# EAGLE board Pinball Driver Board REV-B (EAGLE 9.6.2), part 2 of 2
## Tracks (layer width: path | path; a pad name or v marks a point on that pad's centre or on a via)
+3.3VDC
  Top 1.016: R87.2 52.07,109.86
  Top 2.032: U$1.OUT C46.+ 49.53,109.86 52.07,109.86 179.07,109.86 209.66,140.44 209.66,153.03 | X12.1 209.66,153.03 | X6.1 247.12,153.78 246.38,153.03 | 209.66,153.03 246.38,153.03 | X11.3 296.32,155.99 293.37,153.03 246.38,153.03
+12VDC
  Top 0.406: 45.01,165.33 44.86,165.33 45.01,167.81
  Top 1.016: R73.2 45.01,156.84 | ARDUINO_DUE_MASTER.VIN 299.8,100.97 311.15,112.31 311.15,130.18 324.22,143.25 X26.1
  Top 2.032: X26.1 334.24,148.56 334.24,148.59 | 45.01,167.88 45.01,167.81 45.01,165.33 X25.1 45.01,156.84 42.47,154.31 42.47,121.24 39.34,118.11 C45.+ 38.73,117.48 U$1.IN | X11.5 304.24,167.25 304.8,167.81
  Top 2.54: X8.5 22.22,155.58 X8.6
  Top 5.08: 22.22,155.58 22.22,158.36 31.75,167.88 45.01,167.88 | 45.01,167.81 304.8,167.81 320.11,167.81 334.24,153.67 334.24,148.59
/LATCHSEL0  (via drill 0.35)
  Top 0.406: v224.08,111.68 207.82,111.68 IC8.14
  Bottom 0.406: v224.08,111.68 224.49,111.28 224.49,75.51 226.92,73.08 226.92,53.98 226.11,53.16 221.23,53.16 221.23,60.88 217.17,64.95 IC9.4
/LATCHSEL1
  Top 0.406: IC10.14 207.82,84.45 210.26,82.02 218.8,82.02 220.01,80.8 220.01,62.51 217.17,62.51 IC9.5
/LATCHSEL2
  Top 0.406: IC11.14 207.82,57.23 210.26,59.67 217.17,59.67 IC9.6
/LATCHSEL3  (via drill 0.35)
  Top 0.406: v218.8,34.06 211.89,34.06 207.82,30 IC12.14
  Bottom 0.406: v218.8,34.06 218.8,53.57 219.2,53.98 219.2,55.19 217.17,57.23 IC9.7
/WRITETOCOIL  (via drill 0.35)
  Top 0.406: v218.8,80.39 218.8,74.3 217.17,72.67 IC9.1 | v218.8,104.78 250.09,104.78 ARDUINO_DUE_MASTER.8
  Bottom 0.406: v218.8,104.78 v218.8,80.39
A0  (via drill 0.35)
  Top 0.406: v293.17,106.4 296.01,106.4 296.01,101.52 295.2,100.71 284.63,100.71 284.63,96.65 285.44,95.83 298.45,95.83 ARDUINO_DUE_MASTER.A0 | v293.17,141.35 285.44,149.07 272.03,149.07 v270.81,150.29
  Bottom 0.406: v293.17,141.35 v293.17,106.4 | v270.81,150.29 270.81,159.64 X6.7
A1  (via drill 0.35)
  Top 0.406: v286.26,127.53 v300.48,127.53 | v286.26,141.35 279.35,148.26 268.38,148.26 v267.16,149.48
  Bottom 0.406: v300.48,127.53 300.89,127.13 300.89,95.83 298.45,93.4 ARDUINO_DUE_MASTER.A1 | v286.26,141.35 v286.26,127.53 | v267.16,149.48 267.16,159.64 X6.6
A2  (via drill 0.35)
  Top 0.406: v301.3,141.35 292.35,150.29 v272.44,150.29
  Bottom 0.406: v301.3,141.35 301.3,131.19 299.26,129.16 299.26,127.13 300.08,126.31 300.08,100.31 296.82,97.05 296.82,92.58 298.45,90.96 ARDUINO_DUE_MASTER.A2 | v272.44,150.29 270.41,148.26 263.09,148.26 263.09,159.64 X6.5
A3  (via drill 0.35)
  Top 0.406: v294.79,103.15 290.32,107.62 286.66,107.62 v286.26,107.21 | v283.41,141.35 283.41,141.76 278.54,146.63 260.65,146.63 v259.03,148.26
  Bottom 0.406: v294.79,103.15 295.2,103.15 296.01,102.34 296.01,90.96 298.45,88.52 ARDUINO_DUE_MASTER.A3 | v286.26,107.21 284.23,109.25 284.23,137.69 283.41,138.51 v283.41,141.35 | v259.03,148.26 259.03,159.64 X6.4
A4  (via drill 0.35)
  Top 0.406: v302.92,86.08 298.45,86.08 ARDUINO_DUE_MASTER.A4 | v303.73,129.97 299.26,129.97 298.86,129.56 276.1,129.56 v275.69,129.97 | v275.69,141.35 272.03,145.01 258.22,145.01 v254.96,148.26
  Bottom 0.406: v302.92,86.08 303.33,86.49 303.33,129.56 v303.73,129.97 | v275.69,141.35 v275.69,129.97 | v254.96,148.26 254.96,159.64 X6.3
A5  (via drill 0.35)
  Top 0.406: v294.79,101.93 289.51,101.93 v285.04,106.4 | v282.19,141.35 277.72,145.82 259.03,145.82 255.37,149.48 v251.31,149.48
  Bottom 0.406: v294.79,101.93 294.79,86.89 298.45,83.24 ARDUINO_DUE_MASTER.A5 | v285.04,106.4 283.41,108.03 283.41,137.29 282.19,138.51 v282.19,141.35 | v251.31,149.48 251.31,159.64 X6.2
A6  (via drill 0.35)
  Top 0.406: v284.63,138.91 v302.51,138.91 | v284.63,141.35 284.63,141.76 278.94,147.45 261.47,147.45 258.22,150.7 v233.43,150.7
  Bottom 0.406: v302.51,138.91 302.51,95.02 301.7,94.21 301.7,80.39 300.89,79.58 300.89,76.33 297.64,76.33 296.82,77.14 296.82,78.77 298.45,80.39 ARDUINO_DUE_MASTER.A6 | v284.63,141.35 v284.63,138.91 | v233.43,150.7 233.43,159.64 X12.7
A7  (via drill 0.35)
  Top 0.406: v274.07,128.75 v301.3,128.75 | v274.07,141.35 271.22,144.2 234.64,144.2 v229.77,149.07
  Bottom 0.406: v301.3,128.75 301.7,128.35 301.7,95.43 300.89,94.62 300.89,80.8 298.45,78.36 ARDUINO_DUE_MASTER.A7 | v274.07,141.35 v274.07,128.75 | v229.77,149.07 229.77,159.64 X12.6
A8  (via drill 0.35)
  Top 0.406: v306.17,137.69 288.29,137.69 287.88,138.1 285.44,138.1 285.04,137.69 282.6,137.69 280.98,139.32 237.9,139.32 226.52,150.7 v226.52,151.1
  Bottom 0.406: v306.17,137.69 306.58,137.29 306.58,79.58 301.7,74.7 300.08,74.7 298.45,73.08 ARDUINO_DUE_MASTER.A8 | v226.52,151.1 225.7,151.92 225.7,159.64 X12.5
A9  (via drill 0.35)
  Top 0.406: v289.92,103.15 287.48,105.59 v287.48,106.4 | v287.48,136.88 282.19,136.88 280.57,138.51 237.49,138.51 225.3,150.7 v221.64,150.7
  Bottom 0.406: v289.92,103.15 289.51,102.74 289.51,77.55 289.92,77.14 289.92,70.64 298.45,70.64 ARDUINO_DUE_MASTER.A9 | v287.48,136.88 v287.48,106.4 | v221.64,150.7 221.64,159.64 X12.4
A10  (via drill 0.35)
  Top 0.406: v308.61,68.2 298.45,68.2 ARDUINO_DUE_MASTER.A10 | v308.61,135.66 282.19,135.66 280.16,137.69 237.08,137.69 225.3,149.48 v217.98,149.48
  Bottom 0.406: v308.61,68.2 308.2,68.61 308.2,135.25 v308.61,135.66 | v217.98,149.48 217.98,159.64 X12.3
A11  (via drill 0.35)
  Top 0.406: v307.39,65.76 298.45,65.76 ARDUINO_DUE_MASTER.A11 | v305.36,141.35 306.17,142.16 v306.17,148.26 | v302.11,163.3 216.76,163.3 213.51,160.05 X12.2
  Bottom 0.406: v307.39,65.76 307.39,139.32 v305.36,141.35 | v306.17,148.26 306.17,161.67 304.55,163.3 v302.11,163.3
COIL0
  Bottom 1.905: R1.2 24.13,78.74 | 24.13,78.74 25.4,77.47 Q1.D | 24.13,78.74 24.13,71.75 34.92,60.96 X1.1
COIL1
  Bottom 1.905: R2.2 33.02,78.74 | 33.02,78.74 34.29,77.47 Q2.D | 33.02,78.74 33.02,71.75 39.37,65.41 45.72,65.41 48.52,62.61 X1.2
COIL2
  Bottom 1.905: R3.2 41.91,78.74 | 41.91,78.74 43.18,77.47 Q3.D | 41.91,78.74 41.91,71.75 44.45,69.22 47.62,69.22 52.48,64.36 X1.3
COIL3
  Bottom 1.905: R4.2 50.8,78.74 | 50.8,78.74 52.07,77.47 Q4.D | 50.8,78.74 50.8,71.75 56.51,66.04 56.51,61.03 X1.4
COIL4
  Bottom 1.905: R5.2 59.69,78.74 | 59.69,78.74 60.96,77.47 Q5.D | X1.5 60.4,67.23 59.69,67.95 59.69,78.74
COIL5
  Bottom 1.905: R6.2 68.58,78.74 | 68.58,78.74 69.85,77.47 Q6.D | 68.58,78.74 68.58,71.12 64.36,66.9 X1.6
COIL6
  Bottom 1.905: R7.2 77.47,78.74 | 77.47,78.74 78.74,77.47 Q7.D | 77.47,78.74 77.47,72.39 68.32,63.24 X1.7
COIL7
  Bottom 1.905: R8.2 86.36,78.74 | 86.36,78.74 87.63,77.47 Q8.D | 86.36,78.74 86.36,72.39 74.93,60.96 X1.8
COIL8
  Bottom 1.905: R17.2 96.52,78.74 | 96.52,78.74 97.79,77.47 Q9.D | 96.52,78.74 96.52,71.75 107.31,60.96 X2.1
COIL9
  Bottom 1.905: R18.2 105.41,78.74 | 105.41,78.74 106.68,77.47 Q10.D | 105.41,78.74 105.41,71.75 111.76,65.41 118.11,65.41 120.91,62.61 X2.2
COIL10
  Bottom 1.905: R19.2 114.3,78.74 | 114.3,78.74 115.57,77.47 Q11.D | 114.3,78.74 114.3,71.75 117.07,68.99 120.34,68.99 124.87,64.45 X2.3
COIL11
  Bottom 1.905: R20.2 123.19,78.74 | 123.19,78.74 124.46,77.47 Q12.D | 123.19,78.74 123.19,71.75 128.83,66.11 X2.4
COIL12
  Bottom 1.905: R21.2 132.08,78.74 | 132.08,78.74 133.35,77.47 Q13.D | 132.08,78.74 132.08,67.95 132.79,67.23 X2.5
COIL13
  Bottom 1.905: R22.2 140.97,78.74 | 140.97,78.74 142.24,77.47 Q14.D | X2.6 136.75,66.9 140.97,71.12 140.97,78.74
COIL14
  Bottom 1.905: R23.2 149.86,78.74 | 149.86,78.74 151.13,77.47 Q15.D | X2.7 140.71,63.24 149.86,72.39 149.86,78.74
COIL15
  Bottom 1.905: R24.2 158.75,78.74 | 158.75,78.74 160.02,77.47 Q16.D | 158.75,78.74 158.75,72.39 147.32,60.96 X2.8
COIL16
  Bottom 1.905: R33.2 24.13,24.77 | 24.13,24.77 25.4,23.5 Q17.D | 24.13,24.77 24.13,17.78 34.92,6.98 X3.1
COIL17
  Bottom 1.905: R34.2 33.02,24.77 | 33.02,24.77 34.29,23.5 Q18.D | 33.02,24.77 33.02,17.78 39.37,11.43 46.35,11.43 48.52,9.27 X3.2
COIL18
  Bottom 1.905: R35.2 41.91,24.77 | 41.91,24.77 43.18,23.5 Q19.D | 41.91,24.77 41.91,17.78 44.45,15.24 47.62,15.24 52.48,10.39 X3.3
COIL19
  Bottom 1.905: R36.2 50.8,24.77 | 50.8,24.77 52.07,23.5 Q20.D | 50.8,24.77 50.8,17.78 56.51,12.07 56.51,7.06 X3.4
COIL20
  Bottom 1.905: R37.2 59.69,24.77 | 59.69,24.77 60.96,23.5 Q21.D | 59.69,24.77 59.69,13.97 60.4,13.26 X3.5
COIL21
  Bottom 1.905: R38.2 68.58,24.77 | 68.58,24.77 69.85,23.5 Q22.D | 68.58,24.77 68.58,17.15 64.13,12.7 64.13,7.21 X3.6
COIL22
  Bottom 1.905: R39.2 77.47,24.77 | 77.47,24.77 78.74,23.5 Q23.D | 77.47,24.77 77.47,18.41 68.32,9.27 X3.7
COIL23
  Bottom 1.905: R40.2 86.36,24.77 | 86.36,24.77 87.63,23.5 Q24.D | 86.36,24.77 86.36,19.05 74.3,6.98 X3.8
COIL24
  Bottom 1.905: R58.2 96.52,24.77 | 96.52,24.77 97.79,23.5 Q25.D | 96.52,24.77 96.52,17.78 107.31,6.98 X13.1
COIL25
  Bottom 1.905: R60.2 105.41,24.77 | 105.41,24.77 106.68,23.5 Q26.D | 105.41,24.77 105.41,17.78 111.76,11.43 118.11,11.43 120.91,8.63 X13.2
COIL26
  Bottom 1.905: R62.2 114.3,24.77 | 114.3,24.77 115.57,23.5 Q27.D | 114.3,24.77 114.3,17.78 117.47,14.61 120.01,14.61 124.87,9.75 X13.3
COIL27
  Bottom 1.905: R64.2 123.19,24.77 | 123.19,24.77 124.46,23.5 Q28.D | 123.19,24.77 123.19,17.78 128.91,12.07 128.91,7.06 X13.4
COIL28
  Bottom 1.905: R66.2 132.08,24.77 | 132.08,24.77 133.35,23.5 Q29.D | 132.08,24.77 132.08,13.34 132.79,12.63 X13.5
COIL29
  Bottom 1.905: R68.2 140.97,24.77 | 140.97,24.77 142.24,23.5 Q30.D | 140.97,24.77 140.97,16.51 136.75,12.29 X13.6
COIL30
  Bottom 1.905: R70.2 149.86,24.77 | 149.86,24.77 151.13,23.5 Q31.D | 149.86,24.77 149.86,18.41 140.71,9.27 X13.7
COIL31
  Bottom 1.905: R72.2 158.75,24.77 | 158.75,24.77 160.02,23.5 Q32.D | 158.75,24.77 158.75,18.41 147.32,6.98 X13.8
COIL_GND_0-15
  Bottom 1.905: 90.17,92.71 C8.2 Q8.S | Q1.S C1.2 27.94,92.71 | Q2.S C2.2 36.83,92.71 | Q3.S C3.2 45.72,92.71 | Q4.S C4.2 54.61,92.71 | Q5.S C5.2 63.5,92.71 | Q6.S C6.2 72.39,92.71 | Q7.S C7.2 81.28,92.71 | Q9.S C9.2 100.33,92.71 | Q10.S C10.2 109.22,92.71 | Q11.S C11.2 118.11,92.71 | Q16.S C16.2 162.56,92.71 | Q15.S C15.2 153.67,92.71 | Q14.S C14.2 144.78,92.71 | Q13.S C13.2 135.89,92.71 | Q12.S C12.2 127,92.71
  Bottom 10.16: 162.56,92.71 153.67,92.71 144.78,92.71 135.89,92.71 127,92.71 118.11,92.71 109.22,92.71 100.33,92.71 90.17,92.71 81.28,92.71 72.39,92.71 63.5,92.71 54.61,92.71 45.72,92.71 36.83,92.71 27.94,92.71
  Bottom 7.62: 27.94,92.71 19.68,92.71 17.14,95.25 F1.1A
COIL_GND_16-31
  Bottom 1.905: 27.94,38.73 C17.2 Q17.S | 118.75,38.73 118.11,38.1 C27.2 Q27.S | 135.25,38.73 135.89,38.1 C29.2 Q29.S | Q18.S C18.2 36.83,38.73 | Q19.S C19.2 45.72,38.73 | Q20.S C20.2 54.61,38.73 | Q21.S C21.2 63.5,38.73 | Q22.S C22.2 72.39,38.73 | Q23.S C23.2 81.28,38.73 | Q24.S C24.2 90.17,38.73 | Q25.S C25.2 100.33,38.73 | Q26.S C26.2 109.22,38.73 | Q28.S C28.2 127,38.1 127.63,38.73 | Q30.S C30.2 144.78,38.73 | Q31.S C31.2 153.67,38.73 | Q32.S C32.2 162.56,38.73
  Bottom 10.16: 162.56,38.73 153.67,38.73 144.78,38.73 135.25,38.73 127.63,38.73 118.75,38.73 109.22,38.73 100.33,38.73 90.17,38.73 81.28,38.73 72.39,38.73 63.5,38.73 54.61,38.73 45.72,38.73 36.83,38.73 27.94,38.73
  Bottom 7.62: 27.94,38.73 20.32,38.73 17.14,35.56 F2.1A
COILADDRESS0  (via drill 0.35)
  Top 0.406: v245.62,95.02 245.21,94.62 212.7,94.62 209.86,91.77 202.13,91.77 200.1,89.74 IC10.1
  Bottom 0.406: 202.95,59.26 202.95,38.12 200.1,35.28 IC12.1 | 202.95,59.26 200.1,62.1 IC11.1 | 203.76,88.52 200.91,88.52 200.1,89.33 IC10.1 | 203.76,88.52 203.76,60.07 202.95,59.26 | 203.76,88.52 203.76,115.75 200.91,115.75 200.1,116.56 IC8.1 | v245.62,95.02 245.62,92.99 250.09,88.52 ARDUINO_DUE_MASTER.2
COILADDRESS1  (via drill 0.35)
  Top 0.406: IC12.2 199.69,32.44 196.85,35.28 194,35.28 191.57,37.72 191.57,59.67 199.69,59.67 IC11.2 | v246.84,94.21 246.43,93.8 213.11,93.8 210.26,90.96 204.17,90.96 200.51,87.3 200.1,87.3 IC10.2
  Bottom 0.406: IC11.2 199.69,60.07 198.07,61.7 198.07,62.92 202.95,67.79 202.95,84.05 200.1,86.89 IC10.2 199.69,87.3 198.07,88.93 198.07,90.15 202.95,95.02 202.95,113.31 200.91,113.31 200.1,114.12 IC8.2 | v246.84,94.21 250.09,90.96 ARDUINO_DUE_MASTER.3
COILADDRESS2  (via drill 0.35)
  Top 0.406: 198.07,86.08 199.69,84.45 IC10.3 | 198.07,86.08 v198.07,91.77 198.88,92.58 209.45,92.58 213.11,96.24 v248.46,96.24 | v192.79,57.23 199.69,57.23 IC11.3 | 198.07,86.08 v192.79,86.08
  Bottom 0.406: IC12.3 199.69,30 198.07,31.62 198.07,39.75 202.13,43.81 202.13,55.19 200.1,57.23 IC11.3 | v198.07,91.77 202.13,95.83 202.13,109.65 IC8.3 | v248.46,96.24 248.46,95.02 250.09,93.4 ARDUINO_DUE_MASTER.4 | v192.79,86.08 v192.79,57.23
COILADDRESS3  (via drill 0.35)
  Top 0.406: v221.23,73.89 222.05,74.7 222.05,92.99 247.24,92.99 250.09,95.83 ARDUINO_DUE_MASTER.5
  Bottom 0.406: v221.23,73.89 221.23,71.04 217.98,71.04 217.17,70.23 IC9.2
COILADDRESS4  (via drill 0.35)
  Top 0.406: v217.58,80.8 215.14,80.8 215.14,69.42 217.17,67.39 IC9.3 | v217.58,98.27 250.09,98.27 ARDUINO_DUE_MASTER.6
  Bottom 0.406: v217.58,98.27 v217.58,80.8
COILDATA  (via drill 0.35)
  Top 0.406: v247.24,108.84 207.82,108.84 IC8.13
  Bottom 0.406: IC11.13 204.98,51.94 | 204.98,51.94 204.57,51.54 204.57,30.4 207.42,27.56 IC12.13 | 204.98,79.17 207.42,81.61 IC10.13 | 204.98,51.94 204.98,79.17 | 204.98,79.17 204.57,79.58 204.57,108.03 206.6,108.03 207.42,108.84 IC8.13 | v247.24,108.84 247.24,100.31 248.87,100.31 249.28,100.71 250.09,100.71 ARDUINO_DUE_MASTER.7
D22  (via drill 0.35)
  Top 0.406: v127.76,141.35 128.17,140.94 163.12,140.94 164.74,142.57 202.95,142.57 v204.17,141.35 | v226.52,118.19 v204.17,118.19 | v226.52,79.58 248.06,79.58 249.28,80.8 254.96,80.8 v257,78.77
  Bottom 0.406: v127.76,141.35 127.76,147.85 125.32,150.29 IC3.5 | v204.17,118.19 v204.17,141.35 | v226.52,79.58 v226.52,118.19 | v257,78.77 253.75,75.51 253.75,53.57 252.93,52.76 ARDUINO_DUE_MASTER.22
D23  (via drill 0.35)
  Top 0.406: v202.54,141.35 164.74,141.35 163.52,140.13 124.92,140.13 124.92,142.98 125.73,143.79 134.67,143.79 134.67,146.23 133.05,147.85 IC3.9 | v233.83,124.28 v202.54,124.28 | v239.52,48.69 249.28,48.69 249.68,48.28 250.9,48.28 252.53,49.91 ARDUINO_DUE_MASTER.23
  Bottom 0.406: v202.54,124.28 v202.54,141.35 | v233.83,124.28 234.24,123.88 234.24,53.98 v239.52,48.69
D24  (via drill 0.35)
  Top 0.406: v207.82,153.95 134.67,153.95 133.05,155.58 IC3.12 | v211.48,149.48 216.36,149.48 222.45,143.38 229.77,143.38 v235.05,138.1
  Bottom 0.406: v207.82,153.95 211.48,150.29 v211.48,149.48 | v235.05,138.1 235.05,70.23 235.86,69.42 237.49,69.42 237.49,73.48 240.74,76.73 244.81,76.73 248.06,79.98 258.22,79.98 258.22,74.7 255.37,71.86 255.37,52.76 ARDUINO_DUE_MASTER.24
D25  (via drill 0.35)
  Top 0.406: v206.6,164.11 131.01,164.11 125.32,158.42 IC3.2 | v211.48,148.26 218.39,141.35 v225.3,141.35 | v248.46,49.91 v227.74,49.91
  Bottom 0.406: v206.6,164.11 206.6,152.73 211.07,148.26 v211.48,148.26 | v225.3,141.35 225.3,75.92 227.74,73.48 v227.74,49.91 | v248.46,49.91 248.46,49.51 249.68,48.28 254.96,48.28 254.96,49.91 ARDUINO_DUE_MASTER.25
D26  (via drill 0.35)
  Top 0.406: v187.5,121.03 v127.36,121.03 | v193.19,121.03 194.41,122.25 198.07,122.25 198.48,121.84 245.21,121.84 248.87,125.5 257.4,125.5 268.78,114.12 v268.78,110.87 | v257.81,72.67 v270,72.67
  Bottom 0.406: v127.36,121.03 127.36,125.5 125.32,127.53 IC4.5 | v187.5,121.03 189.94,118.59 193.19,118.59 v193.19,121.03 | v268.78,110.87 268.78,80.39 270,79.17 v270,72.67 | ARDUINO_DUE_MASTER.26 v257.81,72.67
D27  (via drill 0.35)
  Top 0.406: v186.28,125.09 IC4.9 | v186.28,62.51 197.66,62.51 198.88,63.73 v215.14,63.73 | v247.24,51.13 v215.14,51.13
  Bottom 0.406: v186.28,62.51 v186.28,125.09 | v215.14,51.13 v215.14,63.73 | v247.24,51.13 247.24,49.51 249.28,47.47 257.81,47.47 ARDUINO_DUE_MASTER.27
D28  (via drill 0.35)
  Top 0.406: v192.38,129.97 135.48,129.97 133.05,132.41 IC4.12 | v200.51,134.04 v192.38,134.04 | v227.74,127.13 v200.51,127.13 | v228.96,71.86 238.3,71.86 238.71,71.45 243.59,71.45 248.46,76.33 248.46,78.77 249.68,79.98 254.15,79.98 256.59,77.55 259.84,77.55 v260.25,77.95
  Bottom 0.406: v192.38,134.04 v192.38,129.97 | v200.51,127.13 v200.51,134.04 | v227.74,127.13 227.74,74.7 228.96,73.48 v228.96,71.86 | v260.25,77.95 260.25,52.76 ARDUINO_DUE_MASTER.28
D29  (via drill 0.35)
  Top 0.406: v164.34,139.32 129.39,139.32 125.32,135.25 IC4.2 | v168.4,8.05 200.51,8.05 203.35,10.9 217.17,10.9 217.98,11.71 v240.33,11.71 | v237.49,46.25 248.87,46.25 250.09,47.47 257.81,47.47 260.25,49.91 ARDUINO_DUE_MASTER.29
  Bottom 0.406: v164.34,139.32 164.74,138.91 164.74,98.68 168.4,95.02 v168.4,8.05 | v240.33,11.71 240.33,25.12 237.49,27.96 v237.49,46.25
D30  (via drill 0.35)
  Top 0.406: v229.77,82.02 244.81,82.02 245.21,81.61 v247.24,81.61
  Bottom 0.406: v229.77,82.02 229.77,79.98 230.99,78.77 230.99,71.04 230.58,70.64 230.58,42.19 226.11,37.72 IC1.18 | v247.24,81.61 248.06,81.61 248.87,80.8 261.47,80.8 261.47,53.98 262.69,52.76 ARDUINO_DUE_MASTER.30
D31  (via drill 0.35)
  Top 0.406: v247.65,47.47 229.77,47.47 229.77,38.53 228.96,37.72 IC1.17
  Bottom 0.406: v247.65,47.47 248.46,46.66 262.69,46.66 262.69,49.91 ARDUINO_DUE_MASTER.31
D32  (via drill 0.35)
  Top 0.406: v230.99,127.13 285.04,127.13 285.85,126.31 v304.55,126.31 | v295.2,75.11 294.79,74.7 287.88,74.7 284.63,71.45 v265.53,71.45
  Bottom 0.406: v230.99,127.13 230.99,79.98 231.8,79.17 231.8,70.64 231.39,70.23 231.39,37.72 IC1.16 | v304.55,126.31 304.14,125.91 304.14,78.36 301.3,75.51 295.2,75.51 v295.2,75.11 | v265.53,71.45 265.53,52.76 ARDUINO_DUE_MASTER.32
D33
  Top 0.406: IC1.15 231.39,39.75 231.39,45.03 248.87,45.03 250.5,46.66 261.87,46.66 265.12,49.91 ARDUINO_DUE_MASTER.33
D34  (via drill 0.35)
  Top 0.406: v229.36,48.69 v235.86,48.69 | v248.46,101.52 v228.96,101.52 | v252.53,102.74 253.34,101.93 v287.88,101.93 | v285.44,68.2 v288.7,71.45 | v280.98,54.79 280.57,54.38 269.6,54.38 267.97,52.76 ARDUINO_DUE_MASTER.34
  Bottom 0.406: v235.86,48.69 235.86,37.72 IC1.14 | v229.36,48.69 229.77,49.1 229.77,71.04 230.18,71.45 230.18,78.36 228.55,79.98 228.55,101.12 v228.96,101.52 | v248.46,101.52 249.68,102.74 v252.53,102.74 | v287.88,101.93 288.7,101.12 v288.7,71.45 | v285.44,68.2 285.44,59.26 v280.98,54.79
D35
  Top 0.406: IC1.13 239.12,37.72 239.93,38.53 239.93,42.6 247.65,42.6 250.9,45.85 263.91,45.85 267.97,49.91 ARDUINO_DUE_MASTER.35
D36  (via drill 0.35)
  Top 0.406: v232.61,43.81 v241.15,43.81 | v248.46,84.45 v232.21,84.45
  Bottom 0.406: v241.15,43.81 241.15,37.72 IC1.12 | v232.61,43.81 232.61,79.58 231.8,80.39 231.8,84.05 v232.21,84.45 | v248.46,84.45 248.46,82.42 249.28,81.61 262.28,81.61 262.28,76.33 270.41,68.2 270.41,52.76 ARDUINO_DUE_MASTER.36
D37
  Top 0.406: IC1.11 243.99,37.72 251.31,45.03 265.53,45.03 270.41,49.91 ARDUINO_DUE_MASTER.37
D38  (via drill 0.35)
  Top 0.406: v233.02,80.8 233.43,80.39 247.65,80.39 248.87,81.61 260.25,81.61 264.31,77.55 271.63,77.55 v272.03,77.95
  Bottom 0.406: v233.02,80.8 233.43,80.39 233.43,53.16 238.71,47.88 238.71,45.85 254.15,45.85 261.06,38.94 261.06,38.53 261.87,37.72 IC5.18 | v272.03,77.95 272.03,53.57 272.85,52.76 ARDUINO_DUE_MASTER.38
D39
  Bottom 0.406: IC5.17 265.12,37.72 272.85,45.44 272.85,49.91 ARDUINO_DUE_MASTER.39
D40  (via drill 0.35)
  Top 0.406: v301.3,44.22 v276.5,44.22 | v284.23,61.29 v296.82,61.29
  Bottom 0.406: v276.5,44.22 274.07,44.22 267.56,37.72 IC5.16 | v301.3,44.22 301.3,51.54 299.26,53.57 296.82,53.57 v296.82,61.29 | v284.23,61.29 275.69,52.76 ARDUINO_DUE_MASTER.40
D41
  Top 0.406: IC5.15 270,37.72 275.28,43 275.28,49.91 ARDUINO_DUE_MASTER.41
D42  (via drill 0.35)
  Top 0.406: v295.61,39.34 293.98,39.34 289.92,35.28 274.47,35.28 272.44,37.31 IC5.14 | v284.23,59.67 v295.61,59.67
  Bottom 0.406: v295.61,59.67 v295.61,39.34 | v284.23,59.67 278.13,53.57 ARDUINO_DUE_MASTER.42
D43
  Bottom 0.406: ARDUINO_DUE_MASTER.43 278.13,40.56 275.28,37.72 IC5.13
D44  (via drill 0.35)
  Top 0.406: v304.14,42.6 282.6,42.6 277.72,37.72 IC5.12 | v304.14,75.11 303.73,75.51 297.23,75.51 295.61,73.89 289.51,73.89 282.19,66.57 282.19,53.98 280.98,52.76 ARDUINO_DUE_MASTER.44
  Bottom 0.406: v304.14,75.11 v304.14,42.6
D45
  Bottom 0.406: IC5.11 280.16,37.72 280.57,38.12 280.57,49.91 ARDUINO_DUE_MASTER.45
D46  (via drill 0.35)
  Top 0.406: v302.92,74.3 302.51,74.7 297.64,74.7 296.01,73.08 291.95,73.08 283.01,64.14 283.01,52.76 ARDUINO_DUE_MASTER.46
  Bottom 0.406: v302.92,74.3 302.92,39.75 IC6.18
D47
  Top 0.406: IC6.17 305.36,39.75 305.36,45.44 287.88,45.44 283.41,49.91 ARDUINO_DUE_MASTER.47
D48  (via drill 0.35)
  Top 0.406: v293.57,30.4 297.23,34.06 306.98,34.06 306.98,38.53 307.8,39.34 IC6.16 | v289.51,30.4 286.66,27.56 v253.75,27.56 | v250.5,28.37 246.02,32.84 v220.01,32.84 | v220.01,60.48 222.86,63.32 222.86,75.51 v237.9,75.51 | v252.12,121.84 255.37,118.59 v261.06,118.59 | v261.06,83.64 266.75,83.64 268.78,81.61 v268.78,78.77 | v284.23,70.23 v270,70.23
  Bottom 0.406: v289.51,30.4 v293.57,30.4 | v253.75,27.56 252.93,28.37 v250.5,28.37 | v220.01,32.84 220.01,35.69 219.61,36.09 219.61,53.16 220.01,53.57 v220.01,60.48 | v237.9,75.51 240.33,77.95 240.33,111.28 248.46,119.41 248.46,123.47 249.68,124.69 252.12,124.69 v252.12,121.84 | v261.06,83.64 v261.06,118.59 | v268.78,78.77 268.78,71.45 v270,70.23 | v284.23,70.23 285.04,69.42 286.66,69.42 286.66,53.57 285.85,52.76 ARDUINO_DUE_MASTER.48
D49
  Top 0.406: IC6.15 310.24,39.75 306.17,43.81 306.17,46.25 289.51,46.25 285.85,49.91 ARDUINO_DUE_MASTER.49
D50
  Top 0.406: IC6.14 311.45,40.97 311.45,53.57 294.79,53.57 293.98,54.38 289.92,54.38 288.29,52.76 ARDUINO_DUE_MASTER.50
D51  (via drill 0.35)
  Top 0.406: v288.29,41.38 v304.14,41.38
  Bottom 0.406: v304.14,41.38 313.89,41.38 315.52,39.75 IC6.13 | ARDUINO_DUE_MASTER.51 v288.29,41.38
D52  (via drill 0.35)
  Top 0.406: v310.64,99.49 299.26,99.49 298.86,99.09 291.13,99.09 v290.73,99.49 | v292.35,71.86 290.73,70.23 v290.73,65.35
  Bottom 0.406: v310.64,99.49 310.64,68.61 309.02,66.98 309.02,45.85 311.86,45.85 317.96,39.75 IC6.12 | v290.73,99.49 290.32,99.09 290.32,77.95 292.35,75.92 v292.35,71.86 | v290.73,65.35 290.73,52.76 ARDUINO_DUE_MASTER.52
D53  (via drill 0.35)
  Top 0.406: v310.24,47.07 293.98,47.07 291.13,49.91 ARDUINO_DUE_MASTER.53
  Bottom 0.406: v310.24,47.07 313.08,47.07 320.4,39.75 IC6.11
DRIVE0
  Bottom 0.406: X17.1 X4.1 218.55,24.24 223.52,29.21 IC1.2
DRIVE1
  Bottom 0.406: X17.2 X4.2 222.51,24.39 226.06,27.94 IC1.3
DRIVE2
  Bottom 0.406: X17.3 X4.3 226.47,24.54 228.6,26.67 IC1.4
DRIVE3
  Bottom 0.406: X17.4 X4.4 231.14,22.94 IC1.5
DRIVE4
  Bottom 0.406: X17.5 X4.5 233.75,22.86 233.75,24.69 233.68,24.77 IC1.6
DRIVE5
  Bottom 0.406: X17.6 X4.6 238.35,24.54 236.22,26.67 IC1.7
DRIVE6
  Bottom 0.406: X17.7 X4.7 242.31,24.39 238.76,27.94 IC1.8
DRIVE7
  Bottom 0.406: X17.8 X4.8 246.27,24.24 241.3,29.21 IC1.9
DRIVE8
  Bottom 0.406: X16.1 X14.1 254.75,24.24 259.71,29.21 IC5.2
DRIVE9
  Bottom 0.406: X16.2 X14.2 258.7,24.39 262.25,27.94 IC5.3
DRIVE10
  Bottom 0.406: X16.3 X14.3 262.67,23.91 264.8,26.04 IC5.4
DRIVE11
  Bottom 0.406: X16.4 X14.4 266.62,24.05 267.33,24.77 IC5.5
DRIVE12
  Bottom 0.406: X16.5 X14.5 270.58,24.05 269.88,24.77 IC5.6
DRIVE13
  Bottom 0.406: X16.6 X14.6 274.55,24.54 272.42,26.67 IC5.7
DRIVE14
  Bottom 0.406: X16.7 X14.7 278.5,24.39 274.95,27.94 IC5.8
DRIVE15
  Bottom 0.406: IC5.9 277.5,29.21 282.46,24.24 X14.8 X16.8
FET0
  Top 0.406: IC8.4 R9.2
FET1
  Top 0.406: R10.2 IC8.5
FET2
  Top 0.406: IC8.6 R11.2
FET3
  Top 0.406: R12.2 IC8.7
FET4
  Top 0.406: R13.2 196.85,99.06 198.12,97.79 206.38,97.79 IC8.9
FET5
  Top 0.406: IC8.10 208.28,101.6 210.19,99.7 210.19,98.43 208.28,96.52 R14.2
FET6
  Top 0.406: IC8.11 211.45,100.33 211.45,97.79 208.92,95.25 195.58,95.25 R15.2
FET7
  Top 0.406: IC8.12 212.73,101.6 212.73,97.16 209.55,93.98 196.85,93.98 R16.2
FET8
  Top 0.406: R25.2 IC10.4
FET9
  Top 0.406: IC10.5 R26.2
FET10
  Top 0.406: R27.2 IC10.6
FET11
  Top 0.406: IC10.7 R28.2
FET12
  Top 0.406: R29.2 196.85,71.75 198.12,70.48 206.38,70.48 IC10.9
FET13
  Top 0.406: IC10.10 208.28,74.3 210.19,72.39 210.19,71.12 208.28,69.22 R30.2
FET14
  Top 0.406: IC10.11 211.45,73.03 211.45,70.48 207.64,66.67 R31.2
FET15
  Top 0.406: IC10.12 212.73,74.3 212.73,69.85 208.28,65.41 195.58,65.41 R32.2
FET16
  Top 0.406: IC11.4 R41.2
FET17
  Top 0.406: R42.2 IC11.5
FET18
  Top 0.406: IC11.6 R43.2
FET19
  Top 0.406: R44.2 IC11.7
FET20
  Top 0.406: R45.2 196.85,44.45 198.12,43.18 206.38,43.18 IC11.9
FET21
  Top 0.406: IC11.10 208.28,46.99 210.19,45.09 210.19,43.81 208.28,41.91 R46.2
FET22
  Top 0.406: IC11.11 211.45,45.72 211.45,43.18 208.92,40.64 195.58,40.64 R47.2
FET23
  Top 0.406: IC11.12 212.73,46.99 212.73,42.55 209.55,39.37 196.85,39.37 R48.2
FET24
  Top 0.406: R57.2 IC12.4
FET25
  Top 0.406: IC12.5 R59.2
FET26
  Top 0.406: R61.2 IC12.6
FET27
  Top 0.406: IC12.7 R63.2
FET28
  Top 0.406: R65.2 196.85,17.15 198.12,15.88 206.38,15.88 IC12.9
FET29
  Top 0.406: IC12.10 208.28,19.69 210.19,17.78 210.19,16.51 208.28,14.61 R67.2
FET30
  Top 0.406: IC12.11 211.45,18.41 211.45,15.88 208.92,13.34 195.58,13.34 R69.2
FET31
  Top 0.406: IC12.12 212.73,19.69 212.73,15.24 209.55,12.07 196.85,12.07 R71.2
GND
  Top 0.406: IC3.1 118.89,160.66 X9.3 | D3.K 243.18,66.57 229.77,53.16 218.39,53.16 217.17,54.38 IC9.8
  Bottom 0.406: IC3.10 127.63,150.5 IC3.4 130.18,158.12 IC3.13 127.63,158.12 IC3.1 | IC4.10 127.63,127.64 IC4.4 130.18,135.25 IC4.13 127.63,135.25 IC4.1 125.09,142.24 | 163.83,144.78 163.83,153.67 | D2.K 239.52,72.67 243.18,69.01 243.18,66.98 D3.K | IC1.19 223.27,37.31 222.45,36.5 222.45,31.62 221.23,30.4 221.23,30 IC1.1 | IC5.19 259.44,37.31 258.62,36.5 258.62,31.22 257.4,30 IC5.1 | IC6.19 300.08,39.34 299.26,38.53 299.26,38.12 298.45,37.31 295.61,37.31 R53.1 | 198.07,144.78 198.07,150.29 S1.4 198.07,150.7 198.07,156.79 S1.3 | 241.96,144.78 241.96,130.38 D4.K | 331.77,75.56 331.77,75.51 334.25,75.51
  Bottom 0.508: 163.83,153.67 D14.K
  Bottom 1.016: 46.35,154.31 D5.K | D6.K 38.73,144.15 37.46,145.41 | C33.- 66.83,151.13 | C37.- 66.83,128.27 | C38.- 83.97,128.27 | C34.- 83.97,151.13 | C35.- 101.11,151.13 | C36.- 118.26,151.13 | C40.- 118.26,128.27 | C39.- 101.11,128.27 | D15.K 48.31,134.57 48.39,134.57 49.48,133.48 49.48,126.42 49.53,126.37 50.8,126.37 51.43,127 | 196.21,71.75 196.21,98.43 196.85,99.06 IC8.8 196.21,99.06 196.21,144.15 | 196.21,71.75 196.21,67.95 | 196.21,67.95 196.21,43.81 | 196.21,43.81 196.21,17.15 | ARDUINO_DUE_MASTER.GND@0 298.45,104.78 | 298.45,104.78 ARDUINO_DUE_MASTER.GND@1 | ARDUINO_DUE_MASTER.GND@4 262.97,120.27 278.47,104.78 278.76,104.78 | 278.76,104.78 298.45,104.78 | 278.82,80.64 278.82,79.35 293.37,64.8 ARDUINO_DUE_MASTER.GND@2 ARDUINO_DUE_MASTER.GND@3 294,49.53 294,38.73 R53.1 294,36.2 R54.1 292.1,34.92 R55.1 290.19,33.66 R56.1 285.12,29.21 | 278.82,80.64 278.82,81.86 278.76,81.92 278.76,104.78 | DUE_SPI.6 278.82,80.64 | C47.2 125.09,142.24 | 118.26,142.24 125.09,142.24 | 196.21,67.95 C48.2 | IC6.10 320.68,33.02 323.21,35.56 R52.1 324.48,36.2 R51.1 326.39,34.92 R50.1 328.29,33.66 R49.1 332.1,33.66 334.25,35.8 334.25,36.2 | IC5.10 285.12,29.84 285.12,29.21 | 196.21,2.29 196.21,17.15 | IC12.8 196.21,17.15 | 214.63,2.29 214.63,23.5 IC1.1 217.17,33.66 IC9.8 | IC1.10 248.92,29.84 | 248.92,29.84 IC5.1 | 248.92,29.84 248.92,2.29 | 125.09,142.24 IC3.7 | IC4.7 125.09,117.48 | IC11.8 196.85,44.45 196.21,43.81 | IC10.8 196.21,71.75 | 196.21,144.15 196.85,144.78 | 196.21,144.78 196.21,144.15 | 285.12,29.21 285.12,2.92 284.48,2.29
  Bottom 10.16: 36.19,145.41 30.48,145.41 14.6,145.41 12.06,145.41 6.1,139.45 6.1,132.72 6.1,125.09 6.1,81.92 6.1,74.93 15.62,65.41 17.14,65.41 | F1.2A 17.14,65.41 | 17.14,65.41 F2.2A
  Bottom 2.032: 36.19,145.41 37.46,145.41 46.35,154.31 48.97,156.92 X25.2 | X9.3 118.26,151.13 118.26,142.24 X21.3 118.26,128.27 118.26,117.48 | X22.3 101.11,151.13 X18.3 101.11,128.27 101.11,117.62 100.97,117.48 | X19.3 83.97,151.13 X23.3 83.97,128.27 83.97,117.62 83.82,117.48 | X7.3 66.83,151.13 X20.3 66.83,128.27 66.83,120.17 64.13,117.48 | X12.8 237.49,159.91 237.49,144.78 | X6.8 274.84,144.78 | X29.2 316.94,75.56 | 316.94,75.56 X27.2 | 166.37,144.78 SD1.16 SD1.15 | SD1.1 SD1.2 184.15,144.78 | C45.- 38.73,127 | 46.35,127 C46.- 44.45,115.57 39.37,110.49 U$1.GND | X11.2 292.36,145.04 292.1,144.78 | X11.4 300.28,145.34 299.72,144.78 | X11.6 308.2,145 307.34,144.15 | X28.2 334.25,83.19 | 316.94,75.56 331.77,75.56 334.25,75.56 | X30.2 334.25,69.22
  Bottom 2.54: X8.3 14.6,155.58 X8.4 | X8.7 30.48,155.58 X8.8 | X26.5 328.93,125.73 X26.6 | X24.4 16.51,132.72 X24.3 X24.2 16.51,125.09 X24.1 | 6.1,81.92 2.29,78.11 2.29,16.07 16.06,2.29 196.21,2.29 214.63,2.29 248.92,2.29 284.48,2.29 331.22,2.29 335.28,6.35 335.28,35.17
  Bottom 5.08: 14.6,155.58 14.6,145.41 | 30.48,155.58 30.48,145.41 30.48,135.25 38.73,127 46.35,127 51.43,127 60.96,117.48 64.13,117.48 83.82,117.48 100.97,117.48 118.26,117.48 125.09,117.48 135.89,117.48 163.19,144.78 163.83,144.78 166.37,144.78 184.15,144.78 196.21,144.78 | 196.85,144.78 198.07,144.78 237.49,144.78 241.96,144.78 274.84,144.78 292.1,144.78 299.72,144.78 306.7,144.78 307.34,144.15 322.58,128.91 322.58,125.73 | 322.58,125.73 322.58,121.29 334.25,109.61 334.25,83.19 334.25,75.56 334.25,75.51 334.25,69.22 334.25,36.2 | 322.58,125.73 328.93,125.73 | 16.51,132.72 6.35,132.72 5.08,133.98 5.08,133.73 6.1,132.72 | 16.51,125.09 6.1,125.09
MAIN_3.3  (via drill 0.35)
  Top 0.406: v295.2,134.44 206.6,134.44 v205.38,133.22 | v205.38,138.91 204.98,139.32 183.03,139.32 181.81,138.1 SD1.4
  Bottom 0.406: SD1.3 181.81,135.25 181.81,137.69 SD1.4 | v295.2,134.44 295.2,114.53 298.45,111.28 ARDUINO_DUE_MASTER.3.3V | v205.38,138.91 v205.38,133.22
MAIN_5  (via drill 0.35)
  Top 0.406: v280.57,79.58 280.16,79.17 272.03,79.17 270.81,80.39 DUE_SPI.2 | v280.57,103.15 283.82,106.4 283.82,108.43 | 283.82,108.43 298.45,108.43 ARDUINO_DUE_MASTER.5V@0 | v247.24,119.81 v191.97,119.81 | v247.24,125.91 247.65,126.31 265.94,126.31 283.82,108.43
  Bottom 0.406: 179.38,135.25 179.38,137.69 SD1.6 | v280.57,103.15 v280.57,79.58 | 179.38,135.25 191.97,122.66 v191.97,119.81 | v247.24,125.91 v247.24,119.81 | 179.38,135.25 SD1.5
MAIN_13
  Top 0.406: R77.2 244.81,117.78 250.09,117.78 ARDUINO_DUE_MASTER.13
MAIN_BD_RX2  (via drill 0.35)
  Top 0.406: v287.48,76.73 v253.34,76.73 | v305.36,98.27 v287.48,98.27 | v304.14,141.35 304.14,155.98 313.08,155.98 316.33,159.23 X11.8
  Bottom 0.406: v253.34,76.73 252.93,76.33 252.93,73.08 250.5,70.64 ARDUINO_DUE_MASTER.17 | v287.48,98.27 v287.48,76.73 | v305.36,98.27 305.76,98.68 305.76,136.47 304.14,138.1 v304.14,141.35
MAIN_BD_RX3  (via drill 0.35)
  Top 0.406: v236.27,70.64 245.21,70.64 250.09,75.51 ARDUINO_DUE_MASTER.15 | v238.3,140.54 238.71,140.13 311.45,140.13 315.93,144.6 v325.68,144.6
  Bottom 0.406: v236.27,70.64 236.68,71.04 236.68,138.91 v238.3,140.54 | v325.68,144.6 325.68,134.44 328.93,131.19 X26.4
MAIN_BD_TX2  (via drill 0.35)
  Top 0.406: v285.85,74.3 251.71,74.3 250.5,73.08 ARDUINO_DUE_MASTER.16 | v285.85,97.05 297.23,97.05 297.64,97.46 304.55,97.46 304.95,97.05 v315.11,97.05 | v312.67,134.04 314.71,136.07 v314.71,141.76
  Bottom 0.406: v285.85,97.05 v285.85,74.3 | v315.11,97.05 315.11,131.6 v312.67,134.04 | v314.71,141.76 312.27,144.2 312.27,159.23 X11.7
MAIN_BD_TX3  (via drill 0.35)
  Top 0.406: v309.42,76.33 294.79,76.33 293.98,75.51 252.93,75.51 250.5,77.95 ARDUINO_DUE_MASTER.14 | v313.89,130.78 318.36,135.25 328.93,135.25 X26.3
  Bottom 0.406: v309.42,76.33 309.42,126.31 v313.89,130.78
MAIN_CS  (via drill 0.35)
  Top 0.406: v211.07,116.56 248.87,116.56 250.09,115.34 ARDUINO_DUE_MASTER.12 | v206.6,140.13 178.56,140.13 176.53,138.1 SD1.8
  Bottom 0.406: SD1.8 SD1.7 | v211.07,116.56 206.6,121.03 v206.6,140.13
MAIN_MISO  (via drill 0.35)
  Top 0.406: v272.85,112.5 v270,109.65 | v272.85,128.35 230.58,128.35 227.74,125.5 v197.66,125.5 | v197.66,131.19 196.85,130.38 193.6,130.38 192.79,131.19 173.28,131.19 169.21,135.25 SD1.13
  Bottom 0.406: SD1.13 169.21,135.25 169.21,137.69 SD1.14 | v270,109.65 270,83.64 270.41,83.24 DUE_SPI.1 | v272.85,128.35 v272.85,112.5 | v197.66,131.19 v197.66,125.5
MAIN_MOSI  (via drill 0.35)
  Top 0.406: v273.25,77.95 273.66,78.36 280.98,78.36 281.79,79.17 281.79,101.12 252.53,101.12 250.9,102.74 v214.32,102.74 | v198.88,123.06 v214.32,123.06 | v198.88,132.82 176.53,132.82 174.09,135.25 SD1.9
  Bottom 0.406: SD1.9 174.09,135.25 174.09,137.69 SD1.10 | v273.25,77.95 273.25,80.39 DUE_SPI.4 | v214.32,123.06 v214.32,102.74 | v198.88,132.82 v198.88,123.06
MAIN_RESET  (via drill 0.35)
  Top 0.406: v275.28,105.99 275.69,106.4 v282.19,106.4 | v282.19,113.31 298.45,113.31 ARDUINO_DUE_MASTER.RESET | v207.82,156.79 202.54,156.79 S1.1 | v213.11,148.26 218.8,142.57 228.96,142.57 235.86,135.66 v280.57,135.66
  Bottom 0.406: S1.2 202.54,150.7 202.54,156.79 S1.1 | v275.28,105.99 275.28,83.24 DUE_SPI.5 | v282.19,106.4 v282.19,113.31 282.19,134.04 v280.57,135.66 | v207.82,156.79 213.11,151.51 v213.11,148.26
MAIN_RX
  Top 0.406: R76.2 246.02,83.24 250.09,83.24 ARDUINO_DUE_MASTER.0
MAIN_SCK  (via drill 0.35)
  Top 0.406: v262.69,118.59 256.59,124.69 249.28,124.69 245.62,121.03 v194.82,121.03 | v194.82,131.6 194.41,132 174.9,132 171.65,135.25 SD1.11
  Bottom 0.406: SD1.11 171.65,135.25 171.65,137.69 SD1.12 | v262.69,118.59 271.22,110.06 271.22,84.86 272.85,83.24 DUE_SPI.3 | v194.82,131.6 v194.82,121.03
MAIN_SD_FAIL  (via drill 0.35)
  Top 0.406: v207.82,141.35 205.79,143.38 160.27,143.38 155.8,147.85 R86.2 | v213.11,112.9 250.09,112.9 ARDUINO_DUE_MASTER.11
  Bottom 0.406: v207.82,141.35 213.11,136.07 v213.11,112.9
MAIN_TX
  Top 0.406: R75.2 241.96,85.67 250.09,85.67 ARDUINO_DUE_MASTER.1
N$1
  Top 0.406: R10.1 183.51,106.05 45.08,106.05 39.37,100.33 39.37,76.2 38.1,74.93 Q2.G
N$3
  Top 0.406: Q1.G 29.37,74.93 30.48,76.04 30.48,100.33 37.46,107.31 182.25,107.31 R9.1
N$4
  Bottom 0.406: R86.1 155.4,155.58 154.58,156.39 154.58,160.45 D14.A
N$5
  Bottom 1.905: R1.1 27.81,100.33 C1.1
N$6
  Bottom 1.905: R2.1 36.7,100.33 C2.1
N$7
  Top 0.406: R11.1 183.51,104.78 52.7,104.78 48.26,100.33 48.26,76.2 46.99,74.93 Q3.G
N$8
  Top 1.016: D15.A 52.07,128.27 R87.1
N$9
  Top 0.406: R41.1 182.88,53.34 37.46,53.34 30.48,46.36 30.48,22.23 29.21,20.96 Q17.G
N$10
  Bottom 1.905: R3.1 45.59,100.33 C3.1
N$12
  Top 0.406: R12.1 182.25,103.51 60.32,103.51 57.15,100.33 57.15,76.2 55.88,74.93 Q4.G
N$14
  Bottom 1.905: R4.1 54.48,100.33 C4.1
N$15
  Top 0.406: R13.1 180.97,102.23 67.94,102.23 66.04,100.33 66.04,76.2 64.77,74.93 Q5.G
N$17
  Bottom 1.905: R5.1 63.37,100.33 C5.1
N$18
  Bottom 1.905: R33.1 27.81,46.36 C17.1
N$19
  Top 0.406: R14.1 176.53,96.52 174.62,98.43 88.27,98.43 74.93,85.09 74.93,76.2 73.66,74.93 Q6.G
N$21
  Bottom 1.905: R6.1 72.26,100.33 C6.1
N$22
  Top 0.406: R42.1 45.08,52.07 39.37,46.36 39.37,22.23 38.1,20.96 Q18.G
N$23
  Top 0.406: R15.1 176.53,93.98 173.35,97.16 95.88,97.16 83.82,85.09 83.82,76.2 82.55,74.93 Q7.G
N$25
  Bottom 1.905: R7.1 81.15,100.33 C7.1
N$26
  Top 0.406: R16.1 176.53,91.44 172.08,95.89 103.5,95.89 92.71,85.09 92.71,76.2 91.44,74.93 Q8.G
N$28
  Bottom 1.905: R8.1 90.04,100.33 C8.1
N$29
  Top 0.406: R25.1 171.45,94.62 112.39,94.62 102.87,85.09 102.87,76.2 101.6,74.93 Q9.G
N$30
  Top 0.406: R75.1 241.96,77.95 241.96,73.08 D2.A
N$31
  Bottom 0.406: R76.1 245.62,75.51 245.62,66.98 D3.A
N$32
  Bottom 1.905: R17.1 100.2,100.33 C9.1
N$33
  Top 0.406: R26.1 170.18,93.34 120.01,93.34 111.76,85.09 111.76,76.2 110.49,74.93 Q10.G
N$34
  Bottom 0.406: R77.1 244.4,125.91 244.4,129.97 D4.A
N$35
  Bottom 1.905: R18.1 109.09,100.33 C10.1
N$36
  Top 0.406: R27.1 168.91,92.08 127.63,92.08 120.65,85.09 120.65,76.2 119.38,74.93 Q11.G
N$38
  Bottom 1.905: R19.1 117.98,100.33 C11.1
N$39
  Top 0.406: R28.1 167.64,90.81 135.25,90.81 129.54,85.09 129.54,76.2 128.27,74.93 Q12.G
N$41
  Bottom 1.905: R20.1 126.87,100.33 C12.1
N$42
  Top 0.406: R29.1 166.37,89.54 142.88,89.54 138.43,85.09 138.43,76.2 137.16,74.93 Q13.G
N$44
  Bottom 1.905: R34.1 36.7,46.36 C18.1
N$45
  Bottom 1.905: R21.1 135.76,100.33 C13.1
N$46
  Top 0.406: R30.1 165.1,88.27 150.5,88.27 147.32,85.09 147.32,76.2 146.05,74.93 Q14.G
N$48
  Bottom 1.905: R22.1 144.65,100.33 C14.1
N$49
  Top 0.406: R31.1 163.83,87 158.12,87 156.21,85.09 156.21,76.2 154.94,74.93 Q15.G
N$51
  Bottom 1.905: R23.1 153.54,100.33 C15.1
N$52
  Top 0.406: R32.1 173.35,74.93 Q16.G
N$53
  Bottom 1.016: D6.A 48.89,141.6 52.7,145.41 R74.1
N$54
  Bottom 1.905: R24.1 162.43,100.33 C16.1
N$55
  Top 0.406: R43.1 182.88,50.8 52.7,50.8 48.26,46.36 48.26,22.23 46.99,20.96 Q19.G
N$56
  Top 1.016: D5.A 51.43,150.5 R73.1
N$57
  Bottom 1.905: R35.1 45.59,46.36 C19.1
N$58
  Top 0.406: R44.1 181.61,49.53 60.96,49.53 57.15,45.72 57.15,22.23 55.88,20.96 Q20.G
N$60
  Bottom 1.905: R36.1 54.48,46.36 C20.1
N$61
  Top 0.406: R45.1 180.34,48.26 68.58,48.26 66.04,45.72 66.04,22.23 64.77,20.96 Q21.G
N$63
  Bottom 1.905: R37.1 63.37,46.36 C21.1
N$64
  Top 0.406: R46.1 176.53,41.91 173.99,44.45 88.27,44.45 74.93,31.12 74.93,22.23 73.66,20.96 Q22.G
N$66
  Bottom 1.905: R38.1 72.26,46.36 C22.1
N$67
  Top 0.406: R47.1 176.53,39.37 172.72,43.18 95.88,43.18 83.82,31.12 83.82,22.23 82.55,20.96 Q23.G
N$69
  Bottom 1.905: R39.1 81.15,46.36 C23.1
N$70
  Top 0.406: R48.1 176.53,36.83 171.45,41.91 103.5,41.91 92.71,31.12 92.71,22.23 91.44,20.96 Q24.G
N$72
  Bottom 1.905: R40.1 90.04,46.36 C24.1
N$73
  Top 0.406: R57.1 170.81,40.64 112.39,40.64 102.87,31.12 102.87,22.23 101.6,20.96 Q25.G
N$74
  Bottom 1.905: R58.1 100.2,46.36 C25.1
N$75
  Top 0.406: R59.1 169.55,39.37 120.01,39.37 111.76,31.12 111.76,22.23 110.49,20.96 Q26.G
N$76
  Bottom 1.905: R60.1 109.09,46.36 C26.1
N$77
  Top 0.406: R61.1 168.27,38.1 127.63,38.1 120.65,31.12 120.65,22.23 119.38,20.96 Q27.G
N$78
  Bottom 1.905: R62.1 117.98,46.36 C27.1
N$79
  Top 0.406: R63.1 167,36.83 135.25,36.83 129.54,31.12 129.54,22.23 128.27,20.96 Q28.G
N$80
  Bottom 1.905: R64.1 126.87,46.36 C28.1
N$81
  Top 0.406: R65.1 165.74,35.56 142.88,35.56 138.43,31.12 138.43,22.23 137.16,20.96 Q29.G
N$82
  Bottom 1.905: R66.1 135.76,46.36 C29.1
N$83
  Top 0.406: R67.1 164.46,34.29 150.5,34.29 147.32,31.12 147.32,22.23 146.05,20.96 Q30.G
N$84
  Bottom 1.905: R68.1 144.65,46.36 C30.1
N$85
  Top 0.406: R69.1 163.19,33.02 158.12,33.02 156.21,31.12 156.21,22.23 154.94,20.96 Q31.G
N$86
  Bottom 1.905: R70.1 153.54,46.36 C31.1
N$87
  Top 0.406: R71.1 172.72,20.96 Q32.G
N$88
  Bottom 1.905: R72.1 162.43,46.36 C32.1
NEOPIXEL0
  Top 0.406: IC3.6 74.93,147.95 62.86,160.02 X7.2
NEOPIXEL1
  Top 0.406: IC3.8 130.18,145.41 126.36,149.22 90.7,149.22 80.25,159.67 80.21,159.64 80.21,161.27 X19.2
NEOPIXEL2
  Top 0.406: IC3.11 127.55,153.03 126.28,151.77 120.65,151.77 117.47,154.94 103.5,154.94 X22.2
NEOPIXEL3
  Top 0.406: IC3.3 118.75,155.58 114.3,160.02 X9.2
NEOPIXEL4
  Top 0.406: IC4.6 74.93,125.09 62.86,137.16 X20.2
NEOPIXEL5
  Top 0.406: IC4.8 130.18,122.56 126.36,126.37 90.8,126.37 80.01,137.16 X23.2
NEOPIXEL6
  Top 0.406: X18.2 103.5,132.08 117.47,132.08 120.65,128.91 131.44,128.91 IC4.11
NEOPIXEL7
  Top 0.406: IC4.3 118.75,132.72 114.3,137.16 X21.2
P  (via drill 0.35)
  Top 0.406: 210.67,35.28 215.14,39.75 215.14,45.03 R88.2 | 210.67,35.28 207.82,32.44 IC12.15 | v253.75,32.03 v291.13,32.03 | 210.67,35.28 v252.93,35.28 | v209.86,78.77 210.67,77.95 v213.92,77.95
  Bottom 0.406: IC8.15 209.86,112.09 209.86,98.68 205.38,94.21 205.38,89.33 207.42,87.3 IC10.15 207.82,86.89 209.86,84.86 v209.86,78.77 | v291.13,32.03 297.64,32.03 IC6.1 | v253.75,32.03 252.93,32.84 v252.93,35.28 | IC11.15 207.82,59.67 209.86,57.63 209.86,39.75 205.38,35.28 205.38,34.47 207.42,32.44 IC12.15 | v213.92,77.95 213.92,46.66 215.14,45.44 R88.2
SENSE0  (via drill 0.35)
  Top 0.406: v299.08,26.04 R56.2
  Bottom 0.406: X15.1 X5.1 297.18,24.02 297.18,24.13 v299.08,26.04 300.36,27.3 IC6.2
SENSE1  (via drill 0.35)
  Top 0.406: R55.2 v302.89,27.3
  Bottom 0.406: X15.2 X5.2 300.99,23.87 300.99,24.13 302.89,26.04 v302.89,27.3 IC6.3
SENSE2  (via drill 0.35)
  Top 0.406: v305.44,28.58 R54.2
  Bottom 0.406: X15.3 X5.3 304.8,23.72 304.8,24.13 305.44,24.77 v305.44,28.58 IC6.4
SENSE3  (via drill 0.35)
  Top 0.406: R53.2 v307.98,29.84
  Bottom 0.406: X15.4 X5.4 307.26,23.42 307.98,24.13 v307.98,29.84 IC6.5
SENSE4  (via drill 0.35)
  Top 0.406: v310.51,29.84 R52.2
  Bottom 0.406: X15.5 X5.5 311.23,23.42 310.51,24.13 v310.51,29.84 IC6.6
SENSE5  (via drill 0.35)
  Top 0.406: v313.06,28.58 R51.2
  Bottom 0.406: X15.6 X5.6 313.69,23.72 313.69,24.13 313.06,24.77 v313.06,28.58 IC6.7
SENSE6  (via drill 0.35)
  Top 0.406: v315.59,27.3 R50.2
  Bottom 0.406: X15.7 X5.7 317.5,23.87 317.5,24.13 315.59,26.04 v315.59,27.3 IC6.8
SENSE7  (via drill 0.35)
  Top 0.406: v319.4,26.04 R49.2
  Bottom 0.406: X15.8 X5.8 321.31,24.02 321.31,24.13 v319.4,26.04 318.13,27.3 IC6.9
VCC  (via drill 0.35)
  Top 1.016: 252.09,2.29 252.09,32.39 IC5.20 | 285.12,2.29 285.12,24.13 297.81,36.83 IC6.20 | R88.1 IC1.20
  Top 2.032: X28.1 325.04,75.56 | 325.04,75.56 X30.1 | X29.1 312.98,75.56 | 312.98,75.56 X27.1 | 312.98,75.56 325.04,75.56 | 325.04,75.56 335.28,75.56
  Top 2.54: X8.1 6.35,155.58 | 6.35,155.58 X8.2 | 6.35,155.58 6.35,153.67 2.29,149.61 2.29,16.51 16.51,2.29 211.45,2.29 | 211.45,2.29 v211.45,5.08 v211.45,6.35 | 211.45,2.29 252.09,2.29 285.12,2.29 331.22,2.29 335.28,6.35 335.28,75.56 335.28,137.16 333.15,139.29 X26.2
  Bottom 1.016: C37.+ 58.9,129.69 X20.1 53.97,138.43 R74.2 | C40.+ 110.34,130.32 X21.1 | C39.+ 93.19,129.69 X18.1 | C38.+ 76.05,129.69 X23.1 | C34.+ 76.05,151.13 | 58.9,151.13 C33.+ | C35.+ 93.19,151.13 | C36.+ 110.34,151.13 | 135.89,167.88 135.89,160.66 | 135.89,160.66 135.89,142.24 132.71,142.24 | v211.45,5.08 v211.45,6.35 211.45,34.92 | 211.45,34.92 211.45,37.47 | 211.45,67.95 211.45,79.38 | 211.45,79.38 217.81,79.38 IC9.16 | C47.1 132.71,142.24 | C48.1 211.45,67.95 | 211.45,67.95 211.45,62.86 | 211.45,62.86 211.45,37.47 | IC3.14 135.89,160.66 | IC4.14 132.71,142.24 | IC8.16 208.92,116.84 211.45,114.3 211.45,89.54 | 211.45,89.54 211.45,79.38 | R88.1 211.45,37.47 | 211.45,34.92 IC12.16 | IC11.16 210.82,62.23 211.45,62.86 | IC10.16 211.45,89.54
  Bottom 2.032: X20.1 58.9,151.13 X7.1 58.9,167.88 | X23.1 76.05,151.13 X19.1 76.05,167.73 76.2,167.88 | X18.1 93.19,151.13 X22.1 93.19,167.4 92.71,167.88 | X21.1 110.34,151.13 X9.1 110.34,167.4 109.85,167.88 | 334.25,147.95 334.25,141.21 332.33,139.29 331.33,139.29 X26.2 | X11.1 288.4,167.77 288.29,167.88
  Bottom 2.54: X8.1 6.98,155.58 X8.2
  Bottom 5.08: 6.98,155.58 6.98,157.72 17.14,167.88 58.9,167.88 | 56.51,167.88 76.2,167.88 92.71,167.88 109.85,167.88 135.89,167.88 288.29,167.88 320.03,167.88 334.25,153.66 334.25,147.95

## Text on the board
tPlace: Backbox Lights | 0 | 1 | 2 | 3 | Reset / Master | "It'll be a day like this one / when the world caves in." | - Switchfoot | SD Failure | A11 - A6 | A5 - A0 | Expansion | 1 | Power Input | 8 | +12V | 4 | 5 | 6 | 7 | +5V | 13 | Coil GND | +3.3V | High Scores | Neopixel Connectors | Kincaid Arcade Pinball Driver Board | Board and design licensed under / CC BY-SA 4.0 | (c) KincaidArcade 8/4/2020 | https://creativecommons.org/ / licenses/by-sa/4.0/ | Designed By: Alexander H. (A 17 year old!) | REV-B | Arduino DUE | Master | TX | RX | 0 | 7 | 8 | 15 | Drive 0-7 | Drive 8-15 | Sense 0-7 | 0 | 7 | 8 | 15 | 0 | 7 | Drive 0-7 | Drive 8-15 | Sense 0-7 | 16 | 23 | 24 | 31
